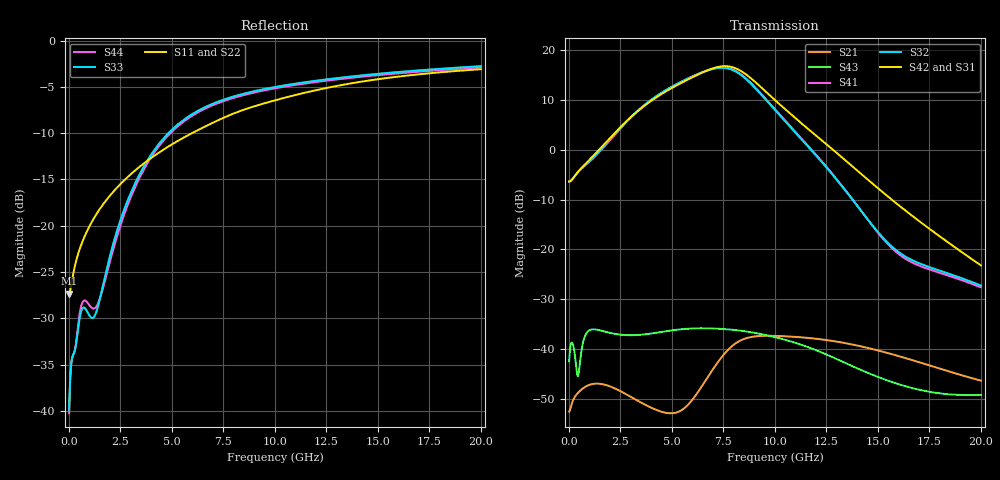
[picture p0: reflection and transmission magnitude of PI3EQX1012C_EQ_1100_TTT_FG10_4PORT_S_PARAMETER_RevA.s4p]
! NPort=4 DATA=2000 NOISE=0 GROUPDELAY=0 COMPLEX_DATAFORMAT=POLAR
! NumOfBlock=1 NumOfParam=0
! .MODEL Smodel S TSTONEFILE=PI3EQX1012C_EQ_1100_TTT_FG10_4PORT_S_PARAMETER_RevA.s4p TYPE=S
!  -- The above .MODEL line can be used for the S element in the netlist.
! The s parameter is extracted from the linear redriver, it is not bi-directional; only s(4,1)s(4,2) and s(3,1)s(3,2)
! should be the insertion loss
!Port definition:
!Port1 = input+
!Port2 = input-
!Port3 = output+
!Port4 = output-
# Hz S MA R  50
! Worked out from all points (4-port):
!   2000 points, 10 MHz to 20 GHz, reference 50 ohm
!   strongest paths, dB at 10 MHz, 5.01 GHz, 10.01 GHz, 15.01 GHz, 20 GHz:
!     S42: -6.4, 12.3, 9.9, -7.8, -23.2
!     S31: -6.4, 12.3, 9.8, -8.0, -23.6
!     S32: -6.4, 12.6, 7.9, -16.6, -27.2
!     S41: -6.4, 12.6, 8.0, -16.7, -27.6
!     S43: -42.4, -36.2, -37.5, -45.5, -49.1
!     S21: -52.4, -52.8, -37.3, -40.2, -46.2
!   lowest |S11| = -27.3 dB at 10 MHz (marker M1), VSWR 1.09, Z = 45.9 - j0.123 ohm
!   |S11| at or under -10 dB: start of sweep to 5.976 GHz
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1e7  0.04301 -178.2  0.002379 1.5  0.0008102 -0.5  0.0008039 -0.5
     0.002388 1.5  0.04109 -178.1  0.000927 -0.5  0.0009197 -0.5
     0.4786 0.3  0.4777 -179.6  0.01016 -4.0  0.007598 -25.7
     0.4773 -179.6  0.4796 0.3  0.007614 -25.8  0.009722 -4.0
4.03e9  0.2339 -124.3  0.002605 1.3  0.0003878 -56.5  0.0003859 -56.8
        0.002593 1.4  0.2374 -123.2  0.0004409 -57.1  0.0004387 -57.5
        3.107 -61.7  3.184 127.1  0.246 -82.9  0.01348 34.6
        3.164 127.8  3.104 -60.0  0.01446 31.6  0.2382 -82.6
5.7e9  0.3045 -123.6  0.002791 51.5  0.00028 -58.3  0.0002789 -59.3
       0.00269 49.3  0.3095 -123.0  0.0003176 -59.3  0.0003164 -60.2
       4.904 -130.3  5.031 58.1  0.3819 -99.0  0.01638 10.3
       5.047 58.4  4.924 -128.4  0.01607 7.6  0.3741 -98.8
6.99e9  0.36 -124.2  0.006655 65.6  0.0002411 -56.0  0.0002391 -57.3
        0.006321 66.3  0.3654 -123.7  0.0002721 -57.2  0.0002699 -58.5
        6.45 165.8  6.397 -6.4  0.4561 -109.1  0.01676 -10.0
        6.448 -6.5  6.486 167.9  0.01621 -10.7  0.4479 -109.0
8.05e9  0.4059 -125.7  0.0117 44.0  0.0002256 -54.3  0.0002227 -55.8
        0.01134 45.5  0.4117 -125.2  0.0002529 -55.6  0.0002497 -57.1
        6.505 101.1  6.112 -71.6  0.5009 -115.6  0.01596 -24.6
        6.182 -72.0  6.544 103.3  0.01565 -24.7  0.4923 -115.4
9.25e9  0.4501 -127.9  0.01383 14.0  0.0002162 -53.8  0.0002123 -55.4
        0.01362 15.5  0.457 -127.4  0.0002407 -55.0  0.0002365 -56.6
        4.317 33.7  3.708 -138.7  0.5403 -121.3  0.01459 -39.1
        3.763 -139.5  4.344 36.3  0.01436 -39.6  0.5316 -121.1
2e10  0.7003 -144.7  0.004941 -75.4  0.0001463 -72.3  0.0001412 -73.8
      0.004872 -74.5  0.7154 -144.4  0.0001622 -72.1  0.0001565 -73.8
      0.06602 101.9  0.04355 28.4  0.7272 -143.5  0.003593 -51.5
      0.04181 26.8  0.06929 106.7  0.003511 -48.8  0.7152 -143.3
